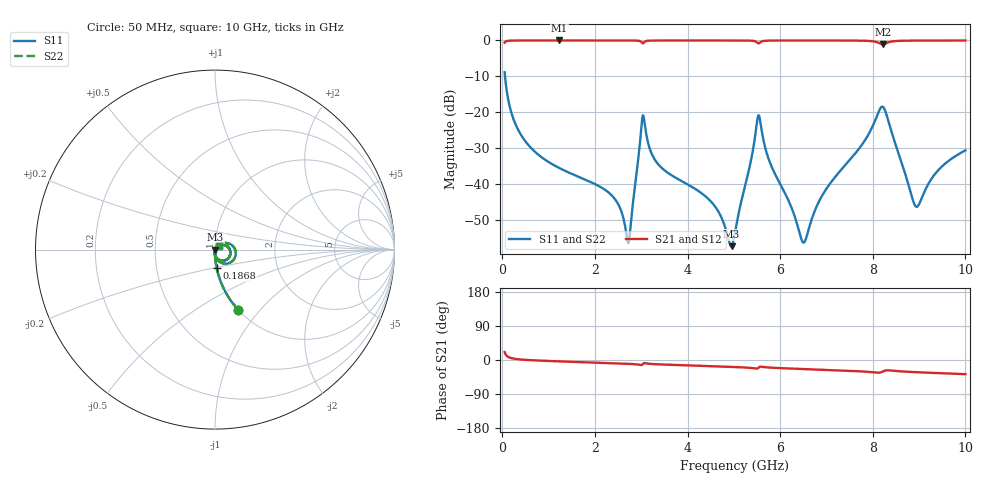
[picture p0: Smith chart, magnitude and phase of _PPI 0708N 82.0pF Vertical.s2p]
! S-Parameter data specifications (vertical orientation):
! Substrate: 40-mil Rogers 3003C, Substrate thickness, H=1.016mm, Dielectric constant, Er=3, Conductor thickness, T_mtl=0.043mm, Loss Tangent, Tand=0.003
! PCB Mounting Pad Footprint: Pad width, PadW=2.54mm , Pad length, PadL=0.51mm , Pad gap, PadG (edge-to-edge)=0.71mm , Reference planes=1.73mm apart
! Created Tue Jan 16 08:54:25 2018
# GHz S MA R 50
! 2 Port Network Data from SP1.SP block
! freq  magS11  angS11  magS21  angS21  magS12  angS12  magS22  angS22
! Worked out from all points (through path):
!   801 points, 50 MHz to 10 GHz, reference 50 ohm
!   highest |S21| = -0.01 dB at 1.232 GHz (marker M1); lowest = -1.1 dB at 8.221 GHz (marker M2)
!   group delay of S21, straight-line fit = 10.9 ps
!   lowest |S11| = -57.3 dB at 4.95 GHz (marker M3), VSWR 1.00, Z = 50.1 - j0.0452 ohm
!   |S11| at or under -10 dB: 58.33 MHz to end of sweep
!   |S22| runs from -57.3 to -8.8 dB; largest |S21 - S12| = 0
!   S11 on the Smith chart (normalised r, x): 50 MHz: 1.00, -0.77; 186.8 MHz: 1.00, -0.21; 10 GHz: 1.04, +0.05
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0.05  0.3611 -69.0  0.9323 21.0  0.9323 21.0  0.3611 -69.0
0.1868125  0.1033 -84.7  0.9945 5.2  0.9945 5.2  0.1033 -84.7
0.5475  0.03588 -89.6  0.9991 0.0  0.9991 0.0  0.03588 -89.6
1.231562  0.01667 -92.3  0.9994 -3.6  0.9994 -3.6  0.01667 -92.3
1.716625  0.01206 -93.4  0.9994 -5.7  0.9994 -5.7  0.01206 -93.4
2.413125  0.006387 -92.1  0.9992 -8.6  0.9992 -8.6  0.006387 -92.1
2.711625  0.001533 -32.3  0.9985 -10.0  0.9985 -10.0  0.001533 -32.3
2.761375  0.002258 27.0  0.9981 -10.3  0.9981 -10.3  0.002258 27.0
3.035  0.09051 -14.4  0.9095 -10.9  0.9095 -10.9  0.09051 -14.4
3.370812  0.01872 -95.7  0.9978 -11.4  0.9978 -11.4  0.01872 -95.7
4.502625  0.005726 -96.2  0.9988 -16.3  0.9988 -16.3  0.005726 -96.2
4.950375  0.00136 -19.4  0.9984 -18.2  0.9984 -18.2  0.00136 -19.4
5.025  0.002124 25.4  0.9983 -18.6  0.9983 -18.6  0.002124 25.4
5.534937  0.09093 -23.6  0.909 -20.0  0.909 -20.0  0.09093 -23.6
5.758813  0.0216 -96.6  0.9946 -19.9  0.9946 -19.9  0.0216 -96.6
6.46775  0.001642 -45.7  0.9982 -23.6  0.9982 -23.6  0.001642 -45.7
6.691625  0.003376 37.9  0.9982 -24.6  0.9982 -24.6  0.003376 37.9
8.221438  0.1185 -27.3  0.8813 -30.0  0.8813 -30.0  0.1185 -27.3
8.345812  0.07216 -70.0  0.9454 -27.3  0.9454 -27.3  0.07216 -70.0
8.942813  0.004801 -22.3  0.9949 -32.2  0.9949 -32.2  0.004801 -22.3
9.403  0.01528 44.7  0.9967 -34.6  0.9967 -34.6  0.01528 44.7
10  0.02943 48.3  0.997 -37.4  0.997 -37.4  0.02943 48.3
